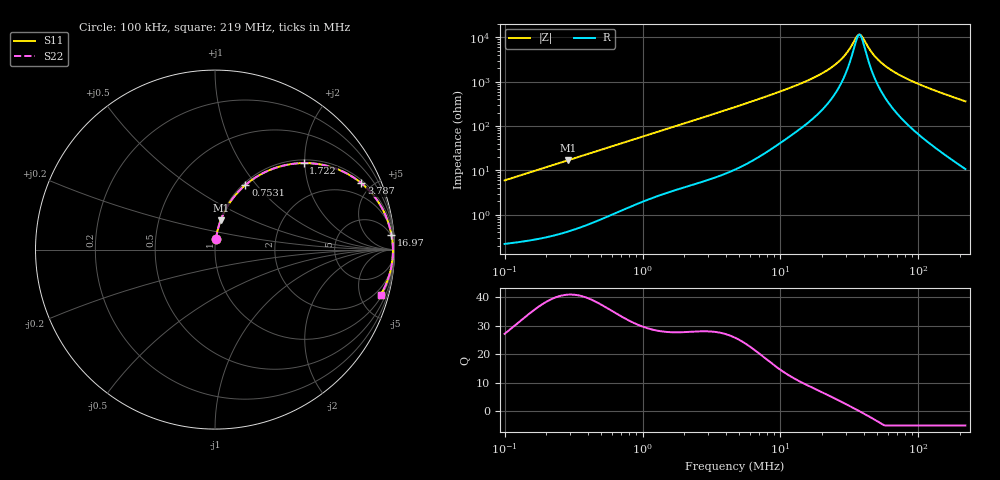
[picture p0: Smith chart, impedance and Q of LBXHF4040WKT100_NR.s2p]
! LBXHF4040WKT100_NR  S-PARAMETER MODEL  ( General Type )
! Model Generated by TAIYO YUDEN Corporation (http://www.ty-top.com)
! Version 1.0
! TAIYO YUDEN Control No. 210719NI43SB-FBB
! Copyright(c) 2021 TAIYO YUDEN CO.,LTD. All Rights Reserved.
! Product Description (link to TY-COMPAS)
! https://ds.yuden.co.jp/TYCOMPAS/or/detail?pn=LBXHF4040WKT100MNR&u=M
! Products Name : Inductors
! Characteristics :
!  Inductance : 10 uH , SRF(min) : 26 MHz , DC Resistance(max) : 0.156 Ohm
!  Rated Current : Saturation :1500 mA , Temp Rise : 1050 mA
!  Case Size : 4.0 x 4.0 / 0.157 x 0.157 [mm/inch] , Thickness : 2 / 0.079 [mm/inch]
!  (Conditions: Temperature = 25 degC , DC Bias Current/Voltage = 0A / 0V)
! External Node Assignments :
!  1  o---GGG---o  2
! GND o---------o GND
! Frequency Range : 0.1MHz  -  218.972167MHz  [ 402 STEP ]
# MHz S RI R 50
! Freq[MHz].  S11 Real  S11 Imag  S21 Real  S21 Imag  S12 Real  S12 Imag  S22 Real  S22 Imag
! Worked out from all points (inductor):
!   401 points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, 100 kHz to 219 MHz, reference 50 ohm
!   read as one part in series: L = 9.44 uH near 103.9 kHz
!   highest Q = 40.8 at 287.9 kHz (marker M1), where L = 9.4 uH
!   self-resonance near 36.62 MHz
!   S11 on the Smith chart (normalised r, x): 100 kHz: 1.00, +0.12; 753.1 kHz: 1.03, +0.88; 1.722 MHz: 1.07, +1.97; 3.787 MHz: 1.16, +4.32; 16.97 MHz: 4, +24; 219 MHz: 1.21, -7.22
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0.1  0.00569 0.059  0.9943 -0.059  0.9943 -0.059  0.00569 0.059
0.287941  0.0319 0.1639  0.9681 -0.1639  0.9681 -0.1639  0.0319 0.1639
0.362673  0.0483 0.2024  0.9517 -0.2024  0.9517 -0.2024  0.0483 0.2024
0.753099  0.1698 0.3603  0.8302 -0.3603  0.8302 -0.3603  0.1698 0.3603
1.315317  0.3701 0.4654  0.6299 -0.4654  0.6299 -0.4654  0.3701 0.4654
1.721646  0.494 0.4822  0.506 -0.4822  0.506 -0.4822  0.494 0.4822
2.433668  0.6533 0.4583  0.3467 -0.4583  0.3467 -0.4583  0.6533 0.4583
3.787335  0.815 0.3704  0.185 -0.3704  0.185 -0.3704  0.815 0.3704
4.770297  0.8728 0.3142  0.1272 -0.3142  0.1272 -0.3142  0.8728 0.3142
9.905636  0.9626 0.1585  0.0374 -0.1585  0.0374 -0.1585  0.9626 0.1585
16.97108  0.9832 0.0816  0.0168 -0.0816  0.0168 -0.0816  0.9832 0.0816
21.79075  0.9878 0.0533  0.0122 -0.0533  0.0122 -0.0533  0.9878 0.0533
26.41082  0.9899 0.0335  0.0101 -0.0335  0.0101 -0.0335  0.9899 0.0335
30.21613  0.9908 0.0202  0.00918 -0.0202  0.00918 -0.0202  0.9908 0.0202
35.92506  0.9914 0.00361  0.00858 -0.00361  0.00858 -0.00361  0.9914 0.00361
37.33357  0.9915 -5.28e-05  0.00853 5.28e-05  0.00853 5.28e-05  0.9915 -5.28e-05
39.55054  0.9915 -0.00556  0.0085 0.00556  0.0085 0.00556  0.9915 -0.00556
44.38725  0.9913 -0.0166  0.00867 0.0166  0.00867 0.0166  0.9913 -0.0166
48.86671  0.991 -0.026  0.00901 0.026  0.00901 0.026  0.991 -0.026
61.54953  0.9893 -0.0497  0.0107 0.0497  0.0107 0.0497  0.9893 -0.0497
101.4729  0.9793 -0.111  0.0207 0.111  0.0207 0.111  0.9793 -0.111
218.9722  0.9223 -0.2533  0.0777 0.2533  0.0777 0.2533  0.9223 -0.2533
